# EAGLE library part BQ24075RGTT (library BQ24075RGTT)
1.5A Li-Ion Charger, Power-Path VQFN16EP BQ24075RGTT, Battery Charge Controller, Lithium-Ion, 4500mA, 16-Pin QFN Source: Datasheet
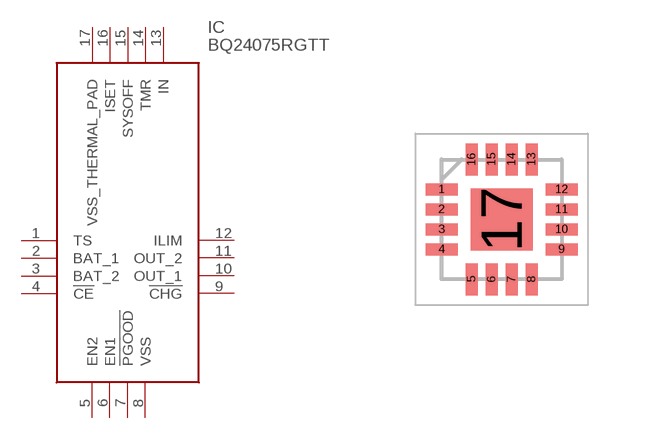
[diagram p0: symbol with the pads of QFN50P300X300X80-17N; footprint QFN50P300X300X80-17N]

Designator prefix IC

## BQ24075RGTT (Arrow_Part_Number: BQ24075RGTT; Arrow_Price/Stock: https://www.arrow.com/en/products/bq24075rgtt/texas-instruments; Description: 1.5A Li-Ion Charger, Power-Path VQFN16EP BQ24075RGTT, Battery Charge Controller, Lithium-Ion, 4500mA, 16-Pin QFN; Height: 0.8mm; Manufacturer_Name: Texas Instruments; Manufacturer_Part_Number: BQ24075RGTT; RS_Part_Number: 8175815P; RS_Price/Stock: http://uk.rs-online.com/web/p/products/8175815P)  [QFN50P300X300X80-17N]
1  TS
2  BAT_1
3  BAT_2
4  !CE
5  EN2
6  EN1
7  !PGOOD
8  VSS  pwr
9  !CHG
10  OUT_1  out
11  OUT_2  out
12  ILIM
13  IN  in
14  TMR
15  SYSOFF
16  ISET
17  VSS_THERMAL_PAD  pwr

## Footprint QFN50P300X300X80-17N (pad centres in mm)
RGT (S-PVQFN-N16)
smd 0.8 x 0.3: 1 -1.5,0.75; 2 -1.5,0.25; 3 -1.5,-0.25; 4 -1.5,-0.75; 9 1.5,-0.75; 10 1.5,-0.25; 11 1.5,0.25; 12 1.5,0.75
smd 0.3 x 0.8: 5 -0.75,-1.5; 6 -0.25,-1.5; 7 0.25,-1.5; 8 0.75,-1.5; 13 0.75,1.5; 14 0.25,1.5; 15 -0.25,1.5; 16 -0.75,1.5
smd 1.55 x 1.55: 17 0,0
